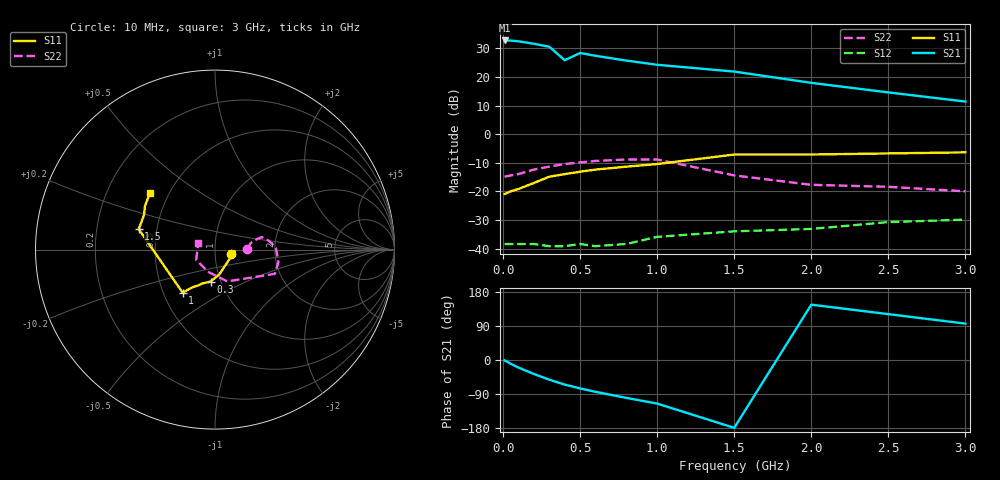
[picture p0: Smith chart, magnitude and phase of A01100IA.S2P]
!  INA-01100  S PARAMETERS
!  Id = 35 mA  LAST UPDATED 11-10-92
# ghz s ma r 50
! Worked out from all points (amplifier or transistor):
!   14 points, 10 MHz to 3 GHz, reference 50 ohm
!   highest |S21| = 32.7 dB at 10 MHz (marker M1)
!   |S21| within 3 dB of that: start of sweep to 317.1 MHz
!   unconditionally stable (mu >= 1): start of sweep to end of sweep
!   at 100 MHz: K = 1.18, MAG = 32.9 dB, |S12| = -38.4 dB
!   at 600 MHz: K = 1.68, MAG = 28.5 dB, |S12| = -39.2 dB
!   at 3 GHz: K = 3.31, MAG = 12.5 dB, |S12| = -29.9 dB
!   S11 on the Smith chart (normalised r, x): 10 MHz: 1.19, -0.06; 300 MHz: 0.89, -0.33; 1 GHz: 0.63, -0.33; 1.5 GHz: 0.39, +0.11; 3 GHz: 0.39, +0.32
0.01  0.09 -16.0  43.4 -1.0  0.012 -1.0  0.18 1.0
0.05  0.1 -27.0  43.1 -10.0  0.012 15.0  0.19 5.0
0.1  0.11 -5.0  41.9 -20.0  0.012 -8.0  0.2 10.0
0.2  0.14 -80.0  38 -37.0  0.012 4.0  0.24 14.0
0.3  0.18 -98.0  33.7 -52.0  0.011 -10.0  0.27 15.0
0.4  0.2 -110.0  19.6 -65.0  0.011 2.0  0.3 10.0
0.5  0.22 -115.0  26.2 -75.0  0.012 -12.0  0.32 6.0
0.6  0.24 -120.0  23.4 -84.0  0.011 -7.0  0.34 1.0
0.8  0.27 -124.0  19.3 -100.0  0.012 -6.0  0.36 -11.0
1  0.3 -127.0  16.3 -115.0  0.016 -5.0  0.36 -22.0
1.5  0.44 165.0  12.4 -179.0  0.02 42.0  0.19 -69.0
2  0.44 154.0  7.88 146.0  0.022 42.0  0.13 -106.0
2.5  0.46 148.0  5.36 121.0  0.029 36.0  0.12 -151.0
3  0.48 139.0  3.71 96.0  0.032 45.0  0.1 159.0
